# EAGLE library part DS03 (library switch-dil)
DIL/CODE SWITCH
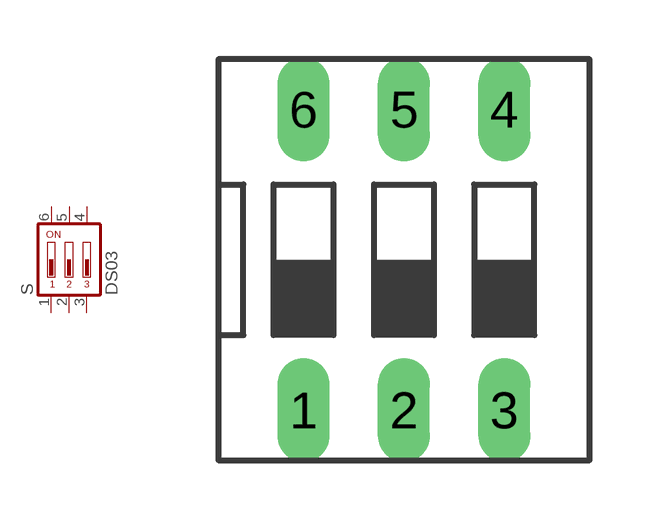
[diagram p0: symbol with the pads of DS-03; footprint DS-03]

Designator prefix S

## DS03 (OC_FARNELL: 1255223; OC_NEWARK: unknown)  [DS-03]
1  1  pas
2  2  pas
3  3  pas
4  4  pas
5  5  pas
6  6  pas

## Footprint DS-03 (pad centres in mm)
DIL/CODE SWITCH Mors distributor Buerklin, 17G552
drill 0.813 long: 1 -2.54,-3.81; 2 0,-3.81; 3 2.54,-3.81; 4 2.54,3.81; 5 0,3.81; 6 -2.54,3.81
